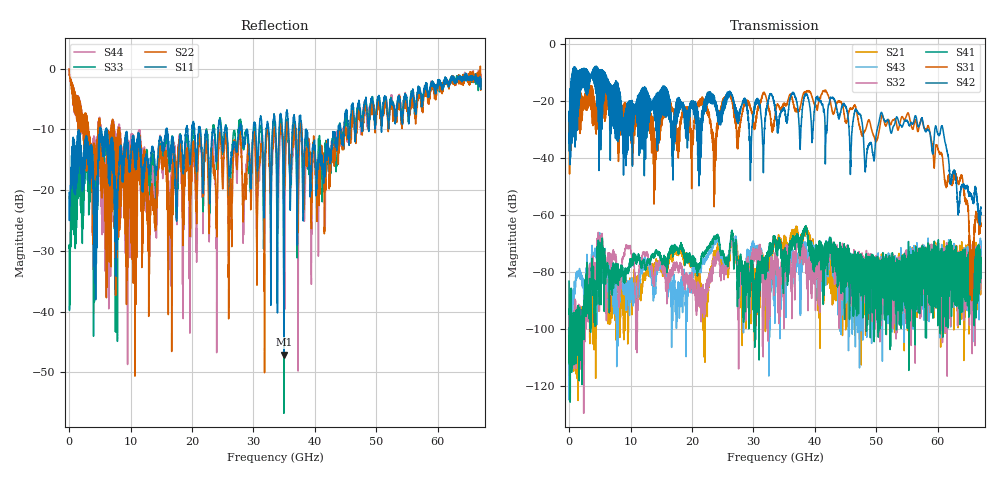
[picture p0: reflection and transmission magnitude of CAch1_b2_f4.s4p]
!Agilent Technologies,N5247A,US51170199,A.09.90.13
!Agilent N5247A: A.09.90.13
!Date: Thursday, October 18, 2018 11:28:32
!Correction: S11(Full 4 Port(1,2,3,4))
!S12(Full 4 Port(1,2,3,4))
!S13(Full 4 Port(1,2,3,4))
!S14(Full 4 Port(1,2,3,4))
!S21(Full 4 Port(1,2,3,4))
!S22(Full 4 Port(1,2,3,4))
!S23(Full 4 Port(1,2,3,4))
!S24(Full 4 Port(1,2,3,4))
!S31(Full 4 Port(1,2,3,4))
!S32(Full 4 Port(1,2,3,4))
!S33(Full 4 Port(1,2,3,4))
!S34(Full 4 Port(1,2,3,4))
!S41(Full 4 Port(1,2,3,4))
!S42(Full 4 Port(1,2,3,4))
!S43(Full 4 Port(1,2,3,4))
!S44(Full 4 Port(1,2,3,4))
!S4P File: Measurements: <S11,S12,S13,S14>,
!<S21,S22,S23,S24>,
!<S31,S32,S33,S34>,
!<S41,S42,S43,S44>:
# Hz S  dB  R 50
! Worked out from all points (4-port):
!   6701 points, 10 MHz to 67 GHz, reference 50 ohm
!   strongest paths, dB at 10 MHz, 16.76 GHz, 33.51 GHz, 50.25 GHz, 67 GHz:
!     S42: -26.9, -30.1, -22.8, -28.7, -57.5
!     S31: -33.5, -23.4, -25.6, -32.5, -62.8
!     S41: -83.2, -71.6, -68.1, -75.4, -74.9
!     S32: -84.1, -79.7, -76.3, -78.7, -74.4
!     S43: -83.3, -98.2, -92.9, -84.9, -83.8
!     S21: -88.0, -75.1, -70.1, -83.6, -78.7
!   lowest |S11| = -47.1 dB at 34.93 GHz (marker M1), VSWR 1.01, Z = 50.3 + j0.304 ohm
!   |S11| at or under -10 dB: start of sweep to 4.986 GHz; 6.095 GHz to 15.8 GHz (9.706 GHz wide, 88.7 % of centre); 38.57 GHz to 43.81 GHz (5.237 GHz wide, 12.7 % of centre)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
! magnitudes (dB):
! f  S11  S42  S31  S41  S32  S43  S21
! 10 MHz  -20.4  -26.9  -33.5  -83.2  -84.1  -83.3  -88.0
! 13.01 GHz  -16.6  -27.4  -23.5  -75.8  -76.3  -75.9  -80.7
! 34.93 GHz  -47.1  -22.3  -21.1  -75.2  -99.8  -78.3  -70.4
! 57.36 GHz  -5.2  -25.9  -26.1  -79.0  -84.3  -75.9  -81.7
! 63.88 GHz  -1.4  -49.4  -46.0  -78.4  -84.7  -85.0  -69.3
! 65.45 GHz  -1.9  -53.0  -76.0  -73.2  -81.7  -78.5  -77.7
! 67 GHz  -3.4  -57.5  -62.8  -74.9  -74.4  -83.8  -78.7
